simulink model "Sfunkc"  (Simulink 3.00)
settings: Solver=ode45  StartTime=0.0  StopTime=2  RelTol=1e-3

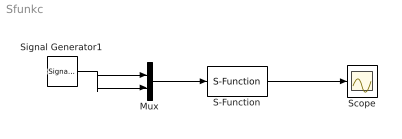
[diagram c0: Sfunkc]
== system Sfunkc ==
  Mux : Mux  Inputs=2
  S-Function : S-Function  FunctionName=Sfunkcija  PortCounts=[]  SFunctionModules=''
  Scope : Scope
  Signal Generator1 : SignalGenerator  WaveForm=sine  Amplitude=1  Frequency=1  Units=Hertz
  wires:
  S-Function/1 -> Scope/1
  Mux/1 -> S-Function/1
  Signal Generator1/1 -> Mux/1, Mux/2
